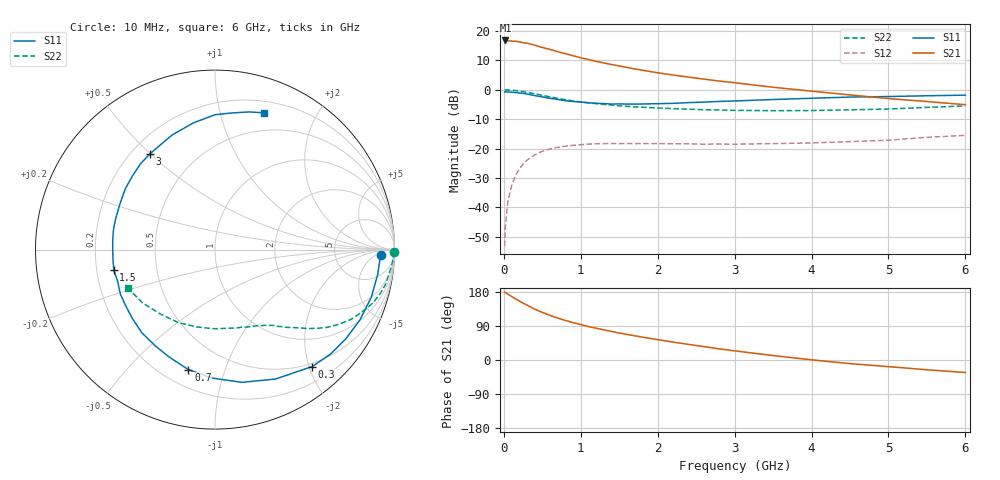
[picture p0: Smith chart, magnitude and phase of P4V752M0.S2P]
! SIEMENS Small Signal Semiconductors
! BFP182
! Si NPN RF Bipolar Junction Transistor in SOT143
! VCE = 0.75 V  IC = 2 mA
! Common Emitter S-Parameters:  March  1996
# GHz  S  MA  R  50
!  f  S11  S21  S12  S22
! GHz  MAG  ANG  MAG  ANG  MAG  ANG  MAG  ANG
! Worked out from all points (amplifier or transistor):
!   36 points, 10 MHz to 6 GHz, reference 50 ohm
!   highest |S21| = 16.7 dB at 20 MHz (marker M1)
!   |S21| within 3 dB of that: start of sweep to 594.8 MHz
!   unconditionally stable (mu >= 1): 2.068 GHz to end of sweep
!   at 250 MHz: K = 0.13, MSG = 20.6 dB, |S12| = -25.2 dB
!   at 1.4 GHz: K = 0.71, MSG = 13.4 dB, |S12| = -18.3 dB
!   at 6 GHz: K = 1.15, MAG = 2.9 dB, |S12| = -15.5 dB
!   S11 on the Smith chart (normalised r, x): 10 MHz: 22, -9; 300 MHz: 0.44, -2.05; 700 MHz: 0.30, -0.76; 1.5 GHz: 0.27, -0.09; 3 GHz: 0.27, +0.50; 6 GHz: 0.31, +1.37
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0.01  0.9249 -1.7  6.767 179.1  0.0022 81.1  0.9946 -0.7
0.02  0.9203 -3.6  6.876 178.2  0.0047 87.3  0.9921 -1.5
0.05  0.9169 -8.9  6.868 173.9  0.0122 85.3  0.992 -3.9
0.1  0.9103 -17.1  6.688 167.9  0.0229 79.7  0.9802 -7.6
0.15  0.8976 -25.9  6.689 161.6  0.0347 74.5  0.9698 -11.5
0.2  0.8822 -34.3  6.51 155.7  0.0448 70.1  0.9525 -14.9
0.3  0.8472 -50.3  6.187 145.0  0.0634 61.0  0.9055 -21.3
0.4  0.7959 -65.0  5.732 134.3  0.0783 52.9  0.8547 -26.9
0.5  0.7545 -78.6  5.224 125.5  0.0898 46.6  0.8048 -31.2
0.6  0.7159 -91.2  4.849 117.8  0.0986 40.8  0.7582 -34.9
0.7  0.6851 -102.5  4.425 110.7  0.1053 36.0  0.7145 -37.9
0.9  0.6312 -121.9  3.784 98.6  0.1138 28.2  0.6459 -42.5
1.1  0.5999 -139.8  3.264 88.2  0.1193 22.5  0.5999 -46.3
1.3  0.5826 -154.8  2.847 79.5  0.1213 17.6  0.5635 -49.5
1.5  0.5754 -168.5  2.538 71.1  0.1213 14.7  0.5333 -52.4
1.8  0.5726 174.0  2.149 60.3  0.122 11.3  0.5051 -56.7
2.2  0.5874 154.5  1.779 47.2  0.1206 8.3  0.4776 -63.3
3  0.6451 124.3  1.317 24.2  0.1189 6.5  0.446 -79.1
3.5  0.6821 110.5  1.102 11.7  0.1215 6.8  0.4411 -90.6
4.5  0.7509 90.1  0.816 -9.6  0.1313 8.0  0.4554 -117.1
5.5  0.7899 76.2  0.631 -25.8  0.1555 8.6  0.5013 -143.8
6  0.8092 70.4  0.557 -33.0  0.1677 5.9  0.531 -156.3
